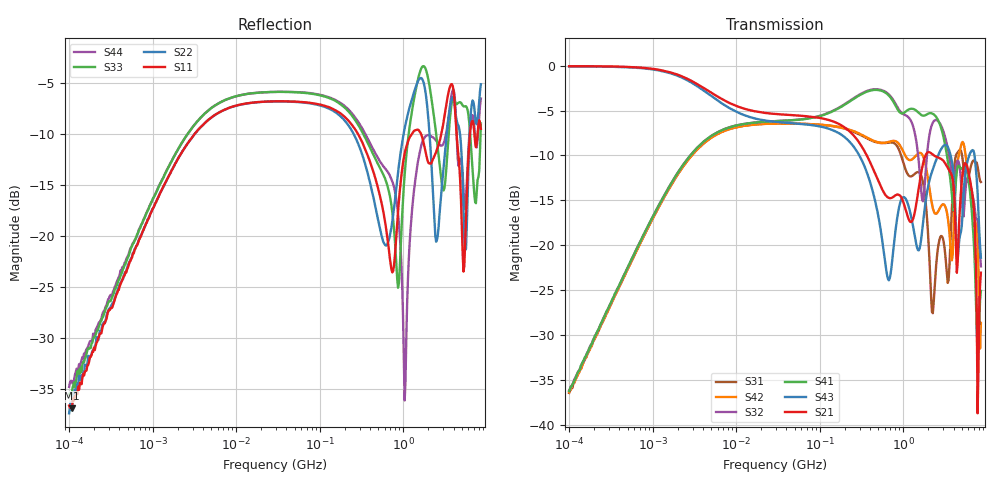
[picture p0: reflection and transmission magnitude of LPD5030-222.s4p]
# MHz S MA R 50
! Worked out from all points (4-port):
!   498 points, 100 kHz to 8.5 GHz, reference 50 ohm
!   strongest paths, dB at 100 kHz, 1.698 MHz, 29.49 MHz, 500.7 MHz, 8.5 GHz:
!     S21: -0.1, -0.8, -5.4, -12.8, -23.1
!     S43: -0.1, -0.9, -6.2, -16.6, -21.4
!     S41: -36.3, -13.0, -6.2, -2.7, -25.1
!     S32: -36.2, -13.0, -6.2, -2.6, -22.4
!     S42: -36.4, -13.2, -6.4, -8.5, -28.7
!     S31: -36.5, -13.2, -6.4, -8.6, -13.0
!   lowest |S11| = -36.9 dB at 107.1 kHz (marker M1), VSWR 1.03, Z = 50.2 + j1.43 ohm
!   |S11| at or under -10 dB: 288 MHz to 1.264 GHz (976.1 MHz wide, 126 % of centre); 1.638 GHz to 2.852 GHz (1.215 GHz wide, 54.1 % of centre); 4.352 GHz to 6.293 GHz (1.941 GHz wide, 36.5 % of centre)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
0.1  0.01481 84.6  0.9934 -0.9  0.01504 -91.0  0.0154 87.6
     0.9934 -0.9  0.01357 84.9  0.0155 87.6  0.01516 -92.7
     0.01504 -91.0  0.0155 87.6  0.01664 75.5  0.991 -1.0
     0.0154 87.6  0.01516 -92.7  0.991 -1.0  0.01831 84.2
0.1070915  0.01436 82.6  0.9934 -0.9  0.01603 -92.0  0.01645 88.5
           0.9934 -0.9  0.01406 86.3  0.01642 87.5  0.01625 -92.7
           0.01603 -92.0  0.01642 87.5  0.01652 79.0  0.9911 -1.1
           0.01645 88.5  0.01625 -92.7  0.9911 -1.1  0.01958 82.0
12.38145  0.4453 11.8  0.5768 -15.5  0.4628 -169.4  0.4736 14.6
          0.5768 -15.5  0.4441 11.6  0.474 14.6  0.4625 -169.6
          0.4628 -169.4  0.474 14.6  0.4951 11.9  0.5313 -18.1
          0.4736 14.6  0.4625 -169.6  0.5313 -18.1  0.495 11.6
296.0887  0.3098 -74.5  0.3742 -85.4  0.4149 79.3  0.6824 -32.3
          0.3742 -85.4  0.2768 -78.2  0.6888 -34.0  0.4194 74.8
          0.4149 79.3  0.6888 -34.0  0.3459 -69.3  0.3179 -90.4
          0.6824 -32.3  0.4194 74.8  0.3179 -90.4  0.3577 -77.8
1039.755  0.2548 -105.4  0.1647 119.9  0.273 -108.0  0.5496 -150.6
          0.1647 119.9  0.3385 -100.3  0.5326 -165.7  0.3198 -103.3
          0.273 -108.0  0.5326 -165.7  0.2007 -75.0  0.1843 -164.9
          0.5496 -150.6  0.3198 -103.3  0.1843 -164.9  0.01569 39.1
1758.138  0.2851 121.6  0.2954 -135.5  0.2128 113.7  0.5268 107.9
          0.2954 -135.5  0.5632 99.5  0.1863 127.4  0.3065 128.2
          0.2128 113.7  0.1863 127.4  0.681 128.1  0.1437 -84.5
          0.5268 107.9  0.3065 128.2  0.1437 -84.5  0.2992 152.1
8500  0.3358 -37.6  0.07036 51.2  0.2251 -16.6  0.05565 28.5
      0.07036 51.2  0.5554 -20.4  0.07628 -83.3  0.03693 1.9
      0.2251 -16.6  0.07628 -83.3  0.3565 -23.3  0.08525 -26.9
      0.05565 28.5  0.03693 1.9  0.08525 -26.9  0.4723 -31.5
